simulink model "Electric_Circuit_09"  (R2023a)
settings: Solver=VariableStepAuto  StartTime=0.0  StopTime=10.0  RelTol=1e-3
libraries: fl_lib x9

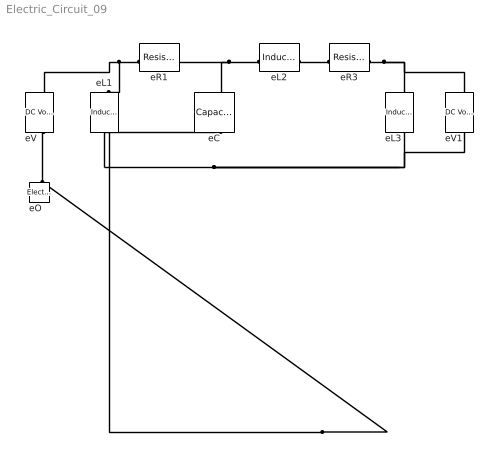
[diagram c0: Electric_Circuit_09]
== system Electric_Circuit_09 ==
  eC : fl_lib/Electrical/Electrical Elements/Capacitor  c=1e-6 F  r=1e-6 Ohm  g=0 1/Ohm  i_specify=off  i_priority=None  i=0 A  i_nominal_specify=off  i_nominal_unit=A  i_nominal_value=1  v_specify=off  v_priority=None  v=0 V  v_nominal_specify=off  v_nominal_unit=V  v_nominal_value=1  vc_specify=off  vc_priority=High  vc=0 V  vc_nominal_specify=off  vc_nominal_unit=V  vc_nominal_value=1
  eL1 : fl_lib/Electrical/Electrical Elements/Inductor  l=1e-6 H  r=0 Ohm  g=1e-9 1/Ohm  i_specify=off  i_priority=None  i=0 A  i_nominal_specify=off  i_nominal_unit=A  i_nominal_value=1  v_specify=off  v_priority=None  v=0 V  v_nominal_specify=off  v_nominal_unit=V  v_nominal_value=1  i_L_specify=off  i_L_priority=High  i_L=0 A  i_L_nominal_specify=off  i_L_nominal_unit=A  i_L_nominal_value=1
  eL2 : fl_lib/Electrical/Electrical Elements/Inductor  l=1e-6 H  r=0 Ohm  g=1e-9 1/Ohm  i_specify=off  i_priority=None  i=0 A  i_nominal_specify=off  i_nominal_unit=A  i_nominal_value=1  v_specify=off  v_priority=None  v=0 V  v_nominal_specify=off  v_nominal_unit=V  v_nominal_value=1  i_L_specify=off  i_L_priority=High  i_L=0 A  i_L_nominal_specify=off  i_L_nominal_unit=A  i_L_nominal_value=1
  eL3 : fl_lib/Electrical/Electrical Elements/Inductor  l=1e-6 H  r=0 Ohm  g=1e-9 1/Ohm  i_specify=off  i_priority=None  i=0 A  i_nominal_specify=off  i_nominal_unit=A  i_nominal_value=1  v_specify=off  v_priority=None  v=0 V  v_nominal_specify=off  v_nominal_unit=V  v_nominal_value=1  i_L_specify=off  i_L_priority=High  i_L=0 A  i_L_nominal_specify=off  i_L_nominal_unit=A  i_L_nominal_value=1
  eO : fl_lib/Electrical/Electrical Elements/Electrical Reference
  eR1 : fl_lib/Electrical/Electrical Elements/Resistor  R=1 Ohm  i_specify=off  i_priority=None  i=0 A  i_nominal_specify=off  i_nominal_unit=A  i_nominal_value=1  v_specify=off  v_priority=None  v=0 V  v_nominal_specify=off  v_nominal_unit=V  v_nominal_value=1
  eR3 : fl_lib/Electrical/Electrical Elements/Resistor  R=1 Ohm  i_specify=off  i_priority=None  i=0 A  i_nominal_specify=off  i_nominal_unit=A  i_nominal_value=1  v_specify=off  v_priority=None  v=0 V  v_nominal_specify=off  v_nominal_unit=V  v_nominal_value=1
  eV : fl_lib/Electrical/Electrical Sources/DC Voltage Source  v0=1 V
  eV1 : fl_lib/Electrical/Electrical Sources/DC Voltage Source  v0=1 V
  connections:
  eO/LConn1 -- eV1/RConn1 -- eL3/RConn1 -- eC/RConn1 -- eL1/RConn1 -- eV/RConn1
  eR1/LConn1 -- eV/LConn1 -- eL1/LConn1
  eL2/LConn1 -- eC/LConn1 -- eR1/RConn1
  eR3/RConn1 -- eV1/LConn1 -- eL3/LConn1
  eR3/LConn1 -- eL2/RConn1
